(* Logix 5000 AddOnInstructionDefinition export ACS_STOP_MOTION; software revision 20.01 *)

ADD_ON_INSTRUCTION ACS_STOP_MOTION   (* revision 2.0, vendor Tolomatic, Inc *)
// Stops ACS Drive Motion
VAR_IN_OUT
   DriveCMD : SINT; {required}   // ACS.O.CMD
END_VAR

ROUTINE Logic   (* ladder *)
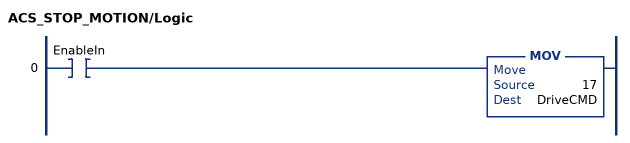
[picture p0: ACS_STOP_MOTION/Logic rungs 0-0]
   0: XIC(EnableIn)MOV(17,DriveCMD);
END_ROUTINE
END_ADD_ON_INSTRUCTION
